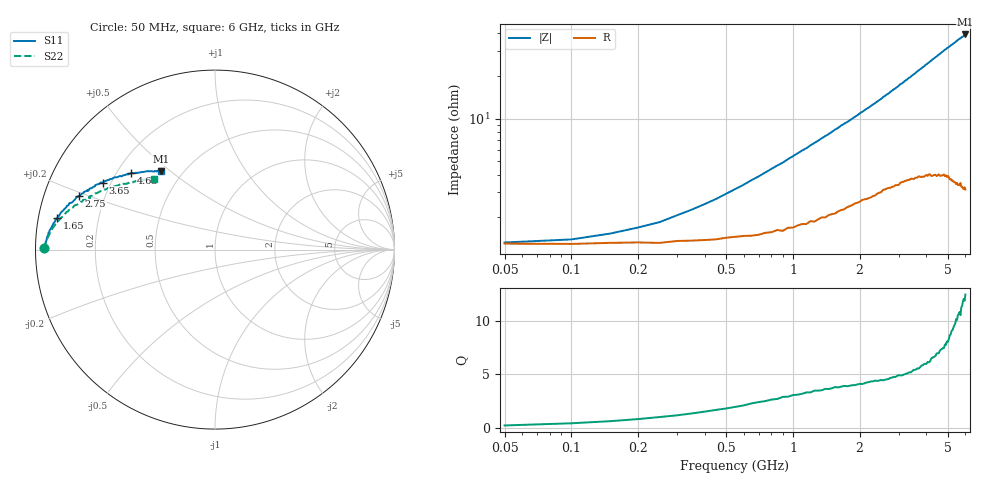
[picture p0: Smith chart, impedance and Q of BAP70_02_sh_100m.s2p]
!	Created	by	janssen	on	Thu	Dec	12	13:21:33	MET	2002
#	HZ	S	MA	R	50
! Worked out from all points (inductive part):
!   120 points, 50 MHz to 6 GHz, reference 50 ohm
!   read as one part in shunt: L = 824 pH near 1 GHz
!   highest Q = 12.5 at 6 GHz (marker M1), where L = 1.04 nH
!   S11 on the Smith chart (normalised r, x): 50 MHz: 0.03, +0.00; 1.65 GHz: 0.05, +0.10; 2.75 GHz: 0.11, +0.19; 3.65 GHz: 0.17, +0.27; 4.65 GHz: 0.26, +0.36; 6 GHz: 0.38, +0.46
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5e7  0.9506 179.6  0.05051 10.6  0.05043 11.3  0.9512 179.6
1e8  0.9494 179.3  0.05305 20.9  0.05335 20.9  0.95 179.2
1.5e8  0.948 178.9  0.05827 29.6  0.05755 29.7  0.9477 178.8
3.5e8  0.9446 177.5  0.08576 50.4  0.08563 50.3  0.9432 177.6
5.5e8  0.9398 176.4  0.1194 59.0  0.1194 59.0  0.9375 176.4
6.5e8  0.9369 175.8  0.1376 61.8  0.1361 61.3  0.9346 175.8
8e8  0.9331 174.8  0.1646 63.9  0.1642 63.5  0.9279 174.9
1.05e9  0.926 173.2  0.2109 65.1  0.2096 64.9  0.9185 173.4
1.4e9  0.9105 170.6  0.2753 65.0  0.2746 64.6  0.9 170.9
1.65e9  0.8967 168.7  0.3222 63.9  0.3188 63.4  0.8828 169.3
2.05e9  0.8715 165.3  0.3929 61.3  0.3893 61.3  0.8563 166.4
2.4e9  0.8482 162.1  0.4535 59.0  0.4492 59.0  0.8252 163.5
2.75e9  0.8153 158.6  0.5124 56.2  0.5067 56.1  0.7943 160.4
3e9  0.797 156.1  0.553 54.2  0.5449 53.9  0.771 158.0
3.05e9  0.7771 154.9  0.5563 53.5  0.5482 53.7  0.7527 157.5
3.1e9  0.7852 155.2  0.5682 53.2  0.5609 53.3  0.7606 157.3
3.65e9  0.7285 149.1  0.646 48.4  0.6355 48.6  0.7029 151.5
4.05e9  0.69 144.3  0.6936 45.1  0.6849 45.5  0.6634 148.0
4.65e9  0.633 137.8  0.7539 40.4  0.7463 41.1  0.6076 142.5
5.05e9  0.598 133.9  0.7844 37.5  0.7781 38.4  0.5765 138.4
5.5e9  0.5627 129.1  0.8153 34.5  0.8116 35.4  0.5495 134.7
6e9  0.5305 124.7  0.8412 31.3  0.8428 32.3  0.5211 130.6
